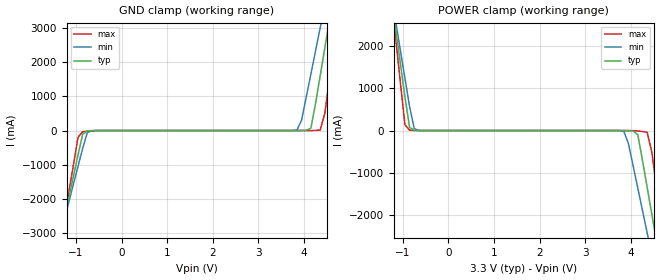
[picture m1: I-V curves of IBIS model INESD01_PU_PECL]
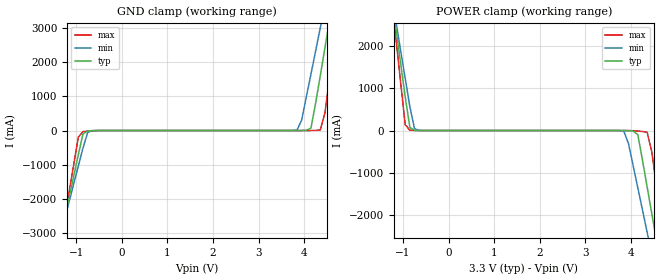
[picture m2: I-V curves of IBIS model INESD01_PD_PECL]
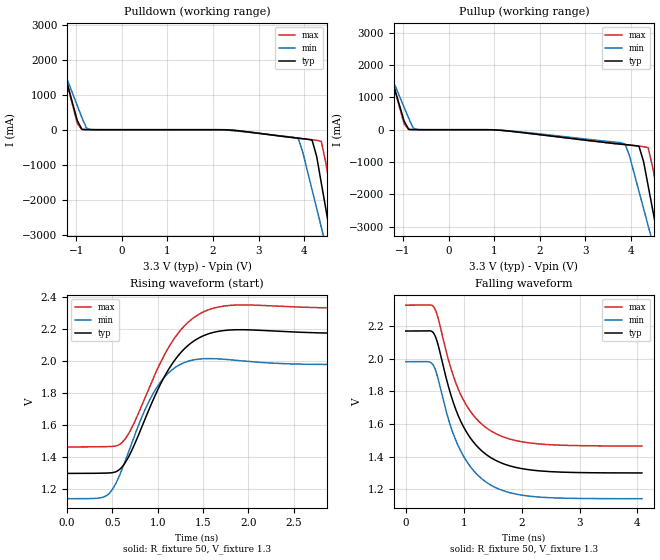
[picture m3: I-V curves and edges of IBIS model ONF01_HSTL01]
|   This file is an IBIS representation of the   |
|   Integrated Device Technology, Inc.   |
|   ICS8633-01   |
|   1-TO-3 DIFFERENTIAL-TO-3.3V LVPECL ZERO DELAY BUFFER   |
[IBIS Ver]   4.1
[File name]   8633_01_3v3.ibs
[File Rev]   1.0
[Date]   19 Mar 2009 | Last modified
|   Apr 26 2007 | Generated
[Source]   Originated at Integrated Devices Technology, Inc.
[Disclaimer]
IDT hereby grants the user of this IBIS model a non-exclusive,
nontransferable license to use this IBIS model under the following terms.
Before using this IBIS model, the user should read this license.
If the user does not accept these terms,  the IBIS model should be
returned to IDT within 30 days.
   The user is granted this license only to use the IBIS model and
is not granted rights to sell, load, rent, lease or license the IBIS
model in whole or in part, or in modified form to anyone other than
user. User may modify the IBIS model to suit its specific
applications but rights to derivative works and such modifications
shall belong to IDT.
   This IBIS model is provided on an "AS IS" basis and IDT makes
absolutely no warranty with respect to the information contained
herein. IDT DISCLAIMS AND CUSTOMER WAIVES ALL WARRANTIES, EXPRESS
OR IMPLIED, INCLUDING WARRANTIES OF MERCHANTABILITY OR FITNESS FOR
A PARTICULAR PURPOSE. The entire risk as to quality and performance
is with the Customer. ACCORDINGLY, IN NO EVENT SHALL THE COMPANY BE
LIABLE FOR ANY DAMAGES, WHETHER IN CONTRACT OR TORT,INCLUDING ANY
LOST PROFITS OR OTHER INCIDENTAL, CONSEQUENTIAL, EXEMPLARY, OR
PUNITIVE DAMAGES ARISING OUT OF THE USE OR APPLICATION OF THE IBIS
model provided in this package. Further, IDT reserves the right to
make changes without notice to any product herein to improve
reliability, function, or design. IDT does not convey any license
under patent rights or any other intellectual property rights,
including those of third parties.
   IDT is not obligated to provide maintenance or support
for the licensed IBIS model.
[Copyright]   Copyright 2007 by Integrated Device Technology, Inc.
[Component]   ICS8633F-01
[Manufacturer] Integrated Devices Technology, Inc.
[Package]
|SSOP 28 Lead
|   typ   min   max
R_pkg   66.7m   54.1m   79.3m
L_pkg   2.262nH   1.601nH   2.922nH
C_pkg   0.329pF   0.232pF   0.427pF
[Pin] signal_name  model_name   R_pin   L_pin   C_pin
1   PLL_SEL   INESD01_PU_PECL   79.3m   2.922n   0.427p
2   VCC   POWER   75.1m   2.702n   0.395p
3   SEL0   INESD01_PD_PECL   70.9m   2.482n   0.362p
4   SEL1   INESD01_PD_PECL   66.7m   2.262n   0.329p
5   CLK0   INESD01_PD_PECL   62.5m   2.041n   0.297p
6   nCLK0   INESD01_PU_PECL   58.3m   1.821n   0.264p
7   CLK1   INESD01_PD_PECL   54.1m   1.601n   0.232p
8   nCLK1   INESD01_PU_PECL   54.1m   1.601n   0.232p
9   CLK_SEL   INESD01_PD_PECL   58.3m   1.821n   0.264p
10   MR   INESD01_PD_PECL   62.5m   2.041n   0.297p
11   VCC   POWER   66.7m   2.262n   0.329p
12   nFB_IN   INESD01_PU_PECL   70.9m   2.482n   0.362p
13   FB_IN   INESD01_PD_PECL   75.1m   2.702n   0.395p
14   VEE   GND   79.3m   2.922n   0.427p
15   VEE   GND   79.3m   2.922n   0.427p
16   nQ0   ONF01_HSTL01   75.1m   2.702n   0.395p
17   Q0   ONF01_HSTL01   70.9m   2.482n   0.362p
18   VCCO   POWER   66.7m   2.262n   0.329p
19   VCCO   POWER   62.5m   2.041n   0.297p
20   nQ1   ONF01_HSTL01   58.3m   1.821n   0.264p
21   Q1   ONF01_HSTL01   54.1m   1.601n   0.232p
22   nQ2   ONF01_HSTL01   54.1m   1.601n   0.232p
23   Q2   ONF01_HSTL01   58.3m   1.821n   0.264p
24   VCCO   POWER   62.5m   2.041n   0.297p
25   VCCO   POWER   66.7m   2.262n   0.329p
26   VEE   GND   70.9m   2.482n   0.362p
27   VEE   GND   75.1m   2.702n   0.395p
28   VCCA   POWER   79.3m   2.922n   0.427p
[Diff Pin]  inv_pin  vdiff tdelay_typ tdelay_min  tdelay_max
|Input
5   6   0.15   0  0  0
7   8   0.15   0  0  0
13   12   0.15   0  0  0
|Output
17   16   NA   0  0  0
21   20   NA   0  0  0
23   22   NA   0  0  0
| Models and submodels in the file (3): INESD01_PU_PECL (Input), INESD01_PD_PECL (Input), ONF01_HSTL01 (Output_ECL)
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[Model]   INESD01_PU_PECL
Model_type  Input
Polarity   Non-Inverting
Vinl = 0.8V
Vinh = 2.0V
|   typ   min   max
C_comp   2pF   1.5pF   2.5pF
|   typ   min   max
[Voltage range]  3.3V   3.15V   3.45V
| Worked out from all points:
|   GND clamp passes 1 mA (typ) near -0.55 V on its own axis
|   POWER clamp passes 1 mA (typ) near -0.67 V on its own axis
[GND_clamp]
|Voltage   I(typ)   I(min)   I(max)
-3.3V     -15.3A     -13.19A    -18.82A
-1.361V   -3.24A     -3.145A    -3.432A
-1.259V   -2.606A    -2.617A    -2.622A
-952.6mV  -705.4mA   -1.038A    -192.5mA
-850.5mV  -99.96mA   -513.6mA   -31.29mA
-646.4mV  -3.852mA   -3.611mA   -8.361mA
3.844V    64.83uA    13.07mA    7.183uA
4.151V    73.26mA    1.652A     800.8uA
4.355V    1.607A     3.003A     15.37mA
4.559V    3.233A     4.356A     1.553A
4.763V    4.861A     5.711A     3.635A
6.6V      19.56A     17.94A     22.42A
[POWER_clamp]
|Voltage   I(typ)   I(min)   I(max)
-3.3V     19.56A     16.84A     24.11A
-1.259V   3.233A     3.262A     3.235A
-1.157V   2.419A     2.586A     2.194A
-952.6mV  795.8mA    1.236A     137.7mA
-850.5mV  73.26mA    563.1mA    8.081mA
-646.4mV  471.5uA    1.942mA    367.2uA
3.844V    -890.5uA   -18.21mA   -111uA
4.151V    -99.96mA   -1.362A    -11.88mA
4.355V    -1.338A    -2.415A    -41.77mA
4.559V    -2.606A    -3.47A     -1.313A
4.763V    -3.875A    -4.526A    -2.933A
6.6V      -15.3A     -14.05A    -17.51A
[Model]   INESD01_PD_PECL
Model_type  Input
Polarity   Non-Inverting
Vinl = 0.8V
Vinh = 2.0V
|   typ   min   max
C_comp   2pF   1.5pF   2.5pF
|   typ   min   max
[Voltage range]  3.3V   3.15V   3.45V
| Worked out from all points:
|   GND clamp passes 1 mA (typ) near -0.55 V on its own axis
|   POWER clamp passes 1 mA (typ) near -0.66 V on its own axis
[GND_clamp]
|Voltage   I(typ)   I(min)   I(max)
-2.586V   -10.86A    -9.487A    -13.15A
-1.361V   -3.24A     -3.145A    -3.432A
-1.259V   -2.606A    -2.617A    -2.622A
-952.6mV  -705.3mA   -1.038A    -192.4mA
-850.5mV  -99.9mA    -513.5mA   -31.23mA
-646.4mV  -3.788mA   -3.549mA   -8.297mA
3.844V    129.1uA    13.13mA    71.12uA
4.151V    73.33mA    1.652A     864.7uA
4.355V    1.607A     3.003A     15.44mA
4.559V    3.233A     4.356A     1.553A
4.763V    4.861A     5.711A     3.635A
5.375V    9.757A     9.783A     9.893A
[POWER_clamp]
|Voltage   I(typ)   I(min)   I(max)
-2.177V   10.57A     9.364A     12.62A
-1.157V   2.42A      2.586A     2.194A
-952.6mV  795.8mA    1.237A     137.8mA
-850.5mV  73.33mA    563.2mA    8.145mA
-646.4mV  535.8uA    2.004mA    431.2uA
3.844V    -826.3uA   -18.14mA   -47.07uA
4.151V    -99.9mA    -1.362A    -11.82mA
4.355V    -1.338A    -2.415A    -41.71mA
4.559V    -2.606A    -3.47A     -1.312A
4.661V    -3.24A     -3.998A    -2.123A
4.763V    -3.875A    -4.526A    -2.933A
5.579V    -8.954A    -8.756A    -9.414A
[Model]   ONF01_HSTL01
Model_type  Output_ECL
Polarity   Non-Inverting
Vmeas = 1.56
Rref = 50
Cref = 0
Vref = 1.3
|   typ   min   max
C_comp   4pF   3.6pF   4.4pF
|   typ   min   max
[Temperature Range]   25   -40   85
|   typ   min   max
[Voltage range]   3.3V   3.135V   3.465V
|   typ   min   max
[Pullup Reference]   3.3V   3.135V   3.465V
|   typ   min   max
[Pulldown Reference]   3.3V   3.135V   3.465V
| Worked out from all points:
|   rising waveform, R_fixture 50, V_fixture 1.3: 20-80 % time 436ps typ, 369ps min, 442ps max; typ from 1.3 V to 2.17 V
|   falling waveform, R_fixture 50, V_fixture 1.3: 20-80 % time 585ps typ, 578ps min, 582ps max; typ from 2.17 V to 1.3 V
| Open source, no load
|  Voltage   I(typ)   I(min)   I(max)
[Pulldown]
-3.3V     11.43A     8.569A     12.06A
-1.583V   3.173A     2.741A     3.273A
-1.482V   2.688A     2.399A     2.757A
-976.5mV  265.3mA    691.7mA    179.8mA
-875.5mV  9.277mA    351.3mA    5.817mA
-673.5mV  497.4uA    4.407mA    311.2uA
3.872V    -242.5mA   -258.2mA   -243.1mA
4.176V    -296.5mA   -1.72A     -288.3mA
4.378V    -1.523A    -2.788A    -338.2mA
4.58V     -3.033A    -3.855A    -1.761A
4.782V    -4.544A    -4.922A    -3.367A
6.6V      -18.28A    -14.6A     -17.98A
|  Voltage   I(typ)   I(min)   I(max)
[Pullup]
-3.3V     11.43A     8.569A     12.06A
-1.785V   4.144A     3.426A     4.306A
-1.583V   3.173A     2.741A     3.273A
-976.5mV  265.3mA    691.7mA    179.8mA
-875.5mV  9.277mA    351.3mA    5.817mA
-673.5mV  497.4uA    4.407mA    311.2uA
3.872V    -459.3mA   -442.5mA   -466.1mA
4.176V    -512mA     -1.904A    -509.8mA
4.378V    -1.738A    -2.972A    -558.7mA
4.58V     -3.247A    -4.039A    -1.98A
4.782V    -4.756A    -5.105A    -3.585A
6.6V      -18.37A    -14.72A    -18.06A
[Ramp]
|   typ   min   max
dV/dt_r   0.716/0.687n   0.698/0.591n   0.708/0.691n
dV/dt_f   0.696/0.94n   0.671/0.923n   0.691/0.935n
R_load =   50.0000
[Rising Waveform]
R_fixture = 50
V_fixture = 1.3   | VCC_typ - 2V
V_fixture_max = 1.465   | VCC_max - 2V
V_fixture_min = 1.135   | VCC_min - 2V
C_fixture = 0.0p
| Time   typ   min   max
0s        1.3V       1.142V     1.465V
427.6ps   1.302V     1.159V     1.467V
612.1ps   1.344V     1.334V     1.496V
731ps     1.465V     1.516V     1.605V
960.6ps   1.774V     1.81V      1.907V
1.121ns   1.95V      1.928V     2.087V
1.301ns   2.081V     1.993V     2.224V
1.522ns   2.163V     2.015V     2.312V
1.805ns   2.194V     2.008V     2.348V
3.867ns   2.17V      1.98V      2.328V
[Falling Waveform]
R_fixture = 50
V_fixture = 1.3   | VCC_typ - 2V
V_fixture_max = 1.465   | VCC_max - 2V
V_fixture_min = 1.135   | VCC_min - 2V
C_fixture = 0.0p
| Time   typ   min   max
0s        2.169V     1.981V     2.328V
395.7ps   2.171V     1.981V     2.329V
485.9ps   2.154V     1.953V     2.315V
559.7ps   2.083V     1.875V     2.247V
760.6ps   1.8V       1.602V     1.963V
941ps     1.623V     1.44V      1.786V
1.183ns   1.483V     1.309V     1.646V
1.482ns   1.391V     1.223V     1.555V
2.257ns   1.315V     1.154V     1.479V
4.077ns   1.3V       1.142V     1.465V
